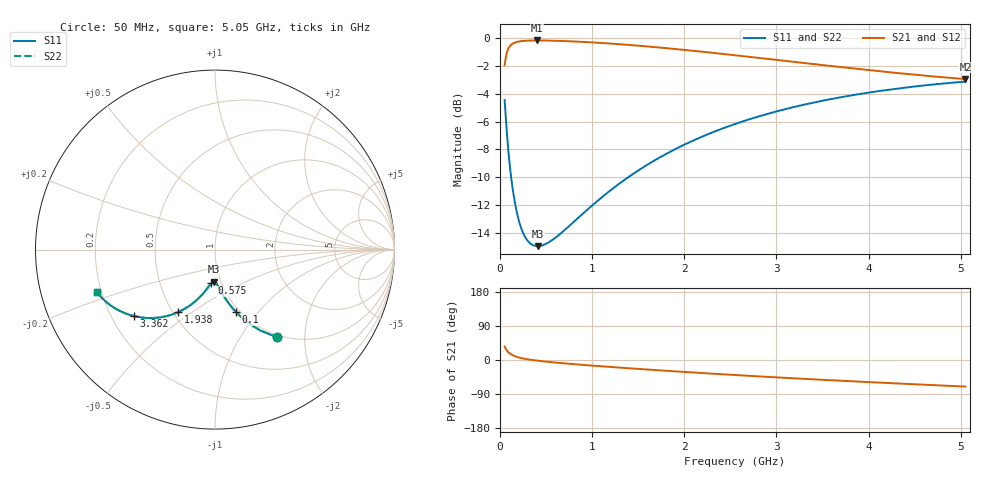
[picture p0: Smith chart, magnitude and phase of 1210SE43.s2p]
! AVX Thin Film Operation		Date: August 2001
! Description: Accu-P® Series, Thin Film, SMD, RF Capacitor
! Part Number: 12101J430FBT
! 50 MHz  -  5.05 GHz
! Serial Measurements
# mhz S db R 50
!	S11		S21		S12		S22
!	dB	Phase	dB	Phase	dB	Phase	dB	Phase
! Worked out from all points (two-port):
!   401 points, 50 MHz to 5.05 GHz, reference 50 ohm
!   highest |S21| = -0.14 dB at 400 MHz (marker M1); lowest = -2.9 dB at 5.05 GHz (marker M2)
!   |S21| within 3 dB of the highest: start of sweep to end of sweep
!   lowest |S11| = -15.0 dB at 412.5 MHz (marker M3), VSWR 1.43, Z = 46.4 - j17.1 ohm
!   |S11| at or under -10 dB: 120.8 MHz to 1.393 GHz (1.272 GHz wide, 168 % of centre)
!   |S22| runs from -15.0 to -3.1 dB; largest |S21 - S12| = 0
!   S11 on the Smith chart (normalised r, x): 50 MHz: 0.96, -1.47; 100 MHz: 0.96, -0.77; 575 MHz: 0.90, -0.35; 1.938 GHz: 0.53, -0.44; 3.362 GHz: 0.29, -0.33; 5.05 GHz: 0.18, -0.17
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50  -4.44 -54.6  -1.94 35.4  -1.94 35.4  -4.44 -54.6
75  -6.86 -65.2  -1.01 24.8  -1.01 24.8  -6.86 -65.2
87.5  -7.86 -68.7  -0.78 21.3  -0.78 21.3  -7.86 -68.7
100  -8.75 -71.5  -0.62 18.4  -0.62 18.4  -8.75 -71.5
125  -10.23 -75.7  -0.43 14.2  -0.43 14.2  -10.23 -75.7
162.5  -11.88 -80.0  -0.29 9.9  -0.29 9.9  -11.88 -80.0
187.5  -12.68 -82.1  -0.24 7.9  -0.24 7.9  -12.68 -82.1
225  -13.58 -84.5  -0.20 5.4  -0.20 5.4  -13.58 -84.5
300  -14.59 -88.1  -0.15 1.8  -0.15 1.8  -14.59 -88.1
400  -14.98 -91.5  -0.14 -1.6  -0.14 -1.6  -14.98 -91.5
412.5  -14.98 -91.9  -0.14 -2.0  -0.14 -2.0  -14.98 -91.9
575  -14.50 -96.1  -0.16 -6.1  -0.16 -6.1  -14.50 -96.1
887.5  -12.71 -102.6  -0.24 -12.7  -0.24 -12.7  -12.71 -102.6
1300  -10.44 -110.1  -0.41 -20.1  -0.41 -20.1  -10.44 -110.1
1725  -8.61 -117.2  -0.65 -27.2  -0.65 -27.2  -8.61 -117.2
1937.5  -7.86 -120.5  -0.78 -30.6  -0.78 -30.6  -7.86 -120.5
2550  -6.17 -129.7  -1.21 -39.7  -1.21 -39.7  -6.17 -129.7
2950  -5.35 -135.2  -1.50 -45.2  -1.50 -45.2  -5.35 -135.2
3362.5  -4.68 -140.5  -1.82 -50.6  -1.82 -50.6  -4.68 -140.5
3387.5  -4.64 -140.9  -1.83 -50.9  -1.83 -50.9  -4.64 -140.9
4225  -3.69 -150.9  -2.44 -61.0  -2.44 -61.0  -3.69 -150.9
5050  -3.11 -160.1  -2.93 -70.1  -2.93 -70.1  -3.11 -160.1
